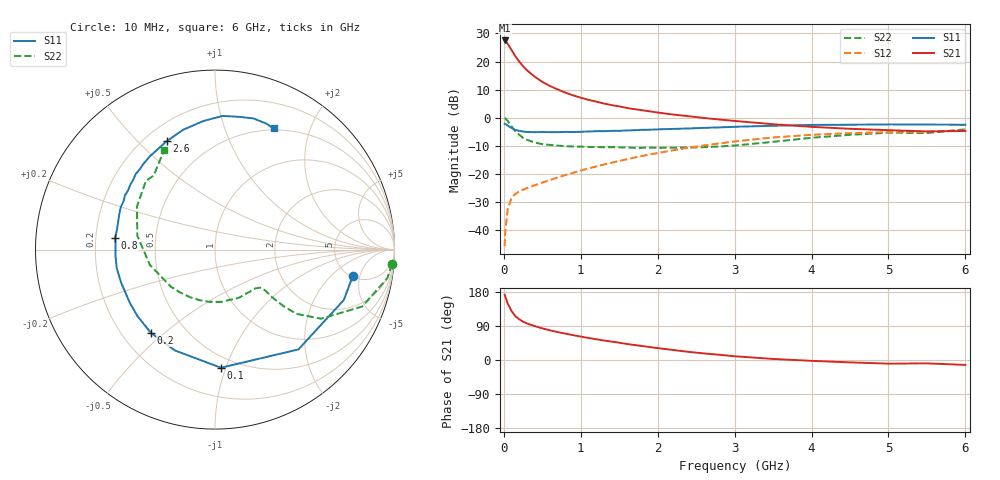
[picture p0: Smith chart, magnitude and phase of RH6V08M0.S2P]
! SIEMENS Small Signal Semiconductors
! BFR106
! Si NPN RF Bipolar Junction Transistor in SOT23
! VCE = 6 V  IC = 8 mA
! Common Emitter S-Parameters:  August  1996
# GHz  S  MA  R  50
!  f  S11  S21  S12  S22
! GHz  MAG  ANG  MAG  ANG  MAG  ANG  MAG  ANG
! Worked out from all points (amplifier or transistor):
!   36 points, 10 MHz to 6 GHz, reference 50 ohm
!   highest |S21| = 27.5 dB at 10 MHz (marker M1)
!   |S21| within 3 dB of that: start of sweep to 91.54 MHz
!   unconditionally stable (mu >= 1): 542.6 MHz to 1.922 GHz; 5.243 GHz to end of sweep
!   at 250 MHz: K = 0.64, MSG = 22.0 dB, |S12| = -25.6 dB
!   at 1.4 GHz: K = 1.10, MAG = 8.3 dB, |S12| = -16.0 dB
!   at 6 GHz: K = 1.01, MAG = -0.8 dB, |S12| = -4.5 dB
!   S11 on the Smith chart (normalised r, x): 10 MHz: 5.13, -3.89; 100 MHz: 0.41, -0.96; 200 MHz: 0.32, -0.45; 800 MHz: 0.28, +0.06; 2.6 GHz: 0.28, +0.61; 6 GHz: 0.48, +1.48
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0.01  0.7816 -10.9  23.7 172.5  0.0052 87.9  0.9888 -4.7
0.02  0.7706 -21.4  23.2 166.8  0.0101 79.3  0.9733 -9.4
0.05  0.7249 -50.1  20.69 149.1  0.0236 66.9  0.88 -21.1
0.1  0.6589 -87.1  16.08 129.2  0.0376 53.0  0.7051 -33.1
0.15  0.6046 -111.7  12.38 115.7  0.0444 47.1  0.577 -38.3
0.2  0.5854 -127.6  9.998 107.6  0.0488 45.5  0.4965 -39.5
0.25  0.5693 -139.3  8.235 101.1  0.0524 45.1  0.4399 -39.8
0.3  0.5595 -148.0  6.988 96.6  0.0562 46.1  0.4068 -39.8
0.4  0.5545 -160.5  5.389 89.5  0.0627 48.7  0.3623 -39.2
0.5  0.5572 -169.3  4.345 83.5  0.0703 51.8  0.3396 -39.2
0.6  0.5553 -176.4  3.669 78.3  0.078 54.2  0.3286 -40.2
0.8  0.5599 173.1  2.8 69.6  0.0958 58.6  0.3121 -43.8
0.9  0.5574 168.3  2.502 65.6  0.1051 60.2  0.3079 -45.8
1.1  0.5693 159.3  2.087 58.2  0.1254 62.1  0.303 -51.9
1.3  0.5763 152.1  1.794 51.5  0.1473 63.0  0.2988 -58.2
1.6  0.5949 142.3  1.491 42.3  0.1832 62.8  0.2951 -69.4
2.2  0.6336 125.1  1.141 26.4  0.2643 58.5  0.2928 -96.3
2.6  0.6612 114.1  0.991 17.4  0.3211 53.4  0.2992 -117.6
3.5  0.7196 95.1  0.767 2.8  0.4458 38.6  0.3728 -166.8
4.5  0.7516 79.8  0.636 -6.3  0.5318 20.2  0.4968 150.9
5.5  0.7579 68.0  0.571 -8.9  0.5644 7.9  0.5359 129.5
6  0.7499 64.2  0.582 -13.0  0.5967 -0.1  0.6219 117.2
